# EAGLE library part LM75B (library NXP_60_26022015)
Digital temperature sensor and thermal watchdog AAL Eindhoven MK
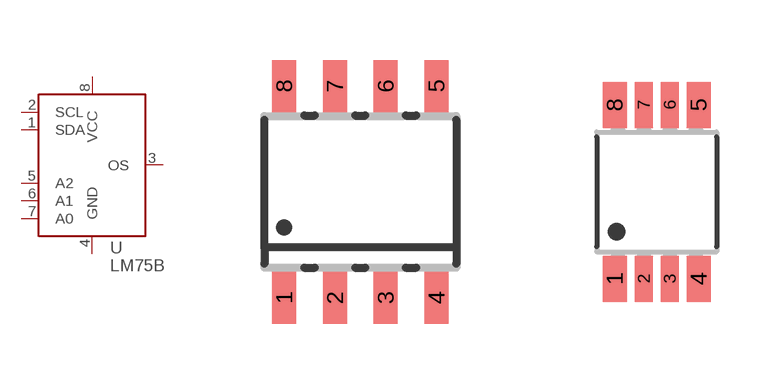
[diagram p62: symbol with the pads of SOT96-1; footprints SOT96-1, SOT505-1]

Designator prefix U

## LM75BD  [SOT96-1]
1  SDA
2  SCL
3  OS  out
4  GND
5  A2  in
6  A1  in
7  A0  in
8  VCC  pwr

## LM75BDP  [SOT505-1]
Pads as for SOT96-1

## LM75BGD  [SOT996-2/3]
Pads as for SOT96-1

## LM75BTP  [SOT1069-2]
Pads as for SOT96-1

## Footprint SOT96-1 (pad centres in mm)
SOT96-1 SO8: plastic small outline package; 8 leads; body width 3.9 mm JEDEC: MS-012 IEC: 076E03
smd 0.6 x 1.3: 1 -1.905,-2.65; 2 -0.635,-2.65; 3 0.635,-2.65; 4 1.905,-2.65; 5 1.905,2.65; 6 0.635,2.65; 7 -0.635,2.65; 8 -1.905,2.65

## Footprint SOT505-1 (pad centres in mm)
SOT505-1 TSSOP8: plastic thin shrink small outline package; 8 leads; body width 3 mm JEDEC: -- IEC: --
smd 0.6 x 1.15: 1 -1.05,-2.175; 4 1.05,-2.175; 5 1.05,2.175; 8 -1.05,2.175
smd 0.45 x 1.15: 2 -0.325,-2.175; 3 0.325,-2.175; 6 0.325,2.175; 7 -0.325,2.175

## Footprint SOT996-2/3 (pad centres in mm)
SOT996-2/3 XSON8U: plastic extremely thin small outline package; no leads;8 terminals; UTLP based; body 3 x 2 x 0.5 mm JEDEC: IEC: -- JEITA: --
smd 0.25 x 1.1: 1 -0.75,-1.45
smd 0.25 x 1: 2 -0.25,-1.5; 3 0.25,-1.5; 4 0.75,-1.5; 5 0.75,1.5; 6 0.25,1.5; 7 -0.25,1.5; 8 -0.75,1.5

## Footprint SOT1069-2 (pad centres in mm)
SOT1069 HWSON8: plastic thermal enhanced very very thin small outline package; no leads;8 terminals; body 2 x 3 x 0.75 mm JEDEC: IEC: -- JEITA: --
smd 0.25 x 0.625: 1 -0.75,-1.413; 2 -0.25,-1.413; 3 0.25,-1.413; 4 0.75,-1.413; 5 0.75,1.413; 6 0.25,1.413; 7 -0.25,1.413; 8 -0.75,1.413
smd 1.6 x 1.6: GP 0,0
